PROGRAM p06_ST_rtrig
VAR
	switch: BOOL;
	light: BOOL;
	button1: BOOL;
	button2: BOOL;
	button: BOOL;
	buttonOld: BOOL;
END_VAR

// Detecting the positive edge on the button
IF button AND NOT buttonOld THEN
	// Detecting the positive edge on the button
	light := NOT light;
	// We omit ELSE to ensure memory retention
END_IF

// Update the old button state
buttonOld := button;

END_PROGRAM
